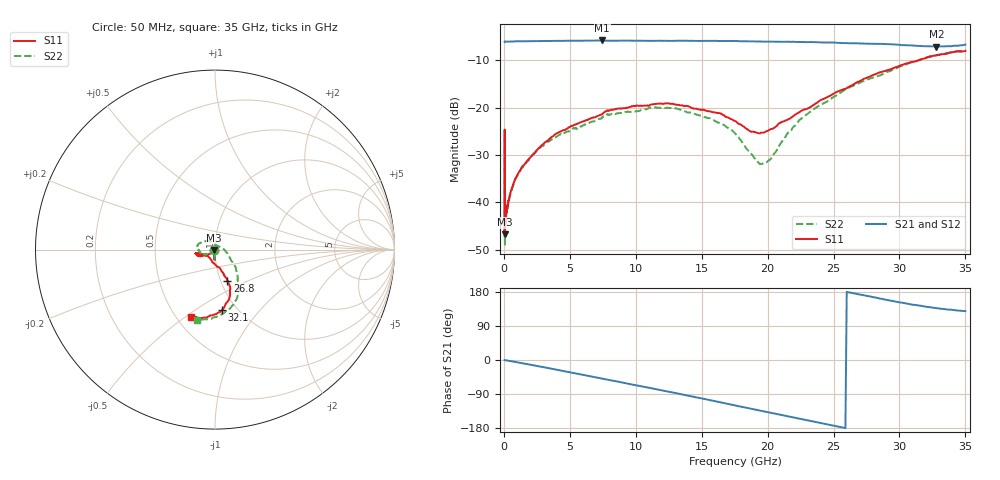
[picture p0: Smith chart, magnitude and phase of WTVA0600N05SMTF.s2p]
! 50 ohm 2-Port S-parameters measured by Modelithics Inc support@modelithics.com  Tampa, FL USA 813-866-6335 (February 2024)
! Smiths Interconnect,  6dB P/N: WTVA0600N05SMTF, Temperature: 25C
! Board: 10 mil Rogers 4350B, Mounting Pad Dimensions: Length: 15 mils, Width: 25 mils, Gap: 40 mils.
# Hz S MA R 50
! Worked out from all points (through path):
!   486 points, 50 MHz to 35 GHz, reference 50 ohm
!   highest |S21| = -5.83 dB at 7.45 GHz (marker M1); lowest = -7.1 dB at 32.8 GHz (marker M2)
!   group delay of S21, straight-line fit = 19.2 ps
!   lowest |S11| = -46.7 dB at 70 MHz (marker M3), VSWR 1.01, Z = 49.6 - j0.209 ohm
!   |S11| at or under -10 dB: start of sweep to 31.47 GHz
!   |S22| runs from -49.2 to -7.9 dB; largest |S21 - S12| = 0.011
!   S11 on the Smith chart (normalised r, x): 50 MHz: 0.99, -0.01; 26.8 GHz: 1.08, -0.38; 32.1 GHz: 0.85, -0.65; 35 GHz: 0.59, -0.52
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5e7  0.004859 -129.8  0.4962 -0.3  0.4961 -0.3  0.004265 -165.5
7e7  0.004617 -152.9  0.4964 -0.4  0.4961 -0.4  0.003764 -143.1
8e7  0.006253 -134.7  0.4966 -0.4  0.496 -0.5  0.003453 -159.5
9e7  0.007693 -163.4  0.4963 -0.5  0.4961 -0.5  0.006326 -159.6
1.1e8  0.006515 -155.8  0.4966 -0.6  0.4963 -0.6  0.005931 -150.3
1.8e8  0.008449 -148.3  0.4966 -1.0  0.4964 -1.0  0.007642 -144.0
5e8  0.01283 -137.2  0.4977 -2.9  0.4976 -2.9  0.01244 -134.1
1.1e9  0.02043 -137.5  0.5002 -6.6  0.5 -6.6  0.02029 -134.4
2.05e9  0.03043 -140.0  0.5022 -12.8  0.5021 -12.8  0.03006 -137.3
3.95e9  0.05286 -146.6  0.506 -25.3  0.5058 -25.3  0.04901 -148.9
5.9e9  0.07085 -151.9  0.5081 -38.3  0.508 -38.3  0.06318 -156.1
7.45e9  0.08536 -154.4  0.5112 -49.1  0.5111 -49.0  0.07923 -163.0
1.17e10  0.1102 -167.4  0.5075 -78.2  0.5074 -78.1  0.09972 171.2
1.57e10  0.0906 -165.8  0.5057 -106.3  0.5058 -106.4  0.07704 142.8
1.76e10  0.07145 -157.2  0.5049 -120.6  0.5048 -120.4  0.05212 120.6
1.97e10  0.05434 -123.7  0.4971 -135.5  0.497 -135.2  0.02596 57.1
2.34e10  0.105 -76.3  0.4915 -162.0  0.4916 -161.7  0.09441 -28.5
2.68e10  0.1855 -68.2  0.4761 174.1  0.4763 174.2  0.1774 -46.7
2.92e10  0.2507 -70.3  0.4669 157.7  0.4668 158.2  0.2408 -57.0
3.21e10  0.3401 -83.6  0.4446 140.2  0.444 141.0  0.3376 -75.5
3.28e10  0.3585 -88.7  0.4413 136.9  0.4414 137.5  0.355 -81.7
3.5e10  0.3962 -109.7  0.4622 128.9  0.462 129.3  0.4037 -104.3
